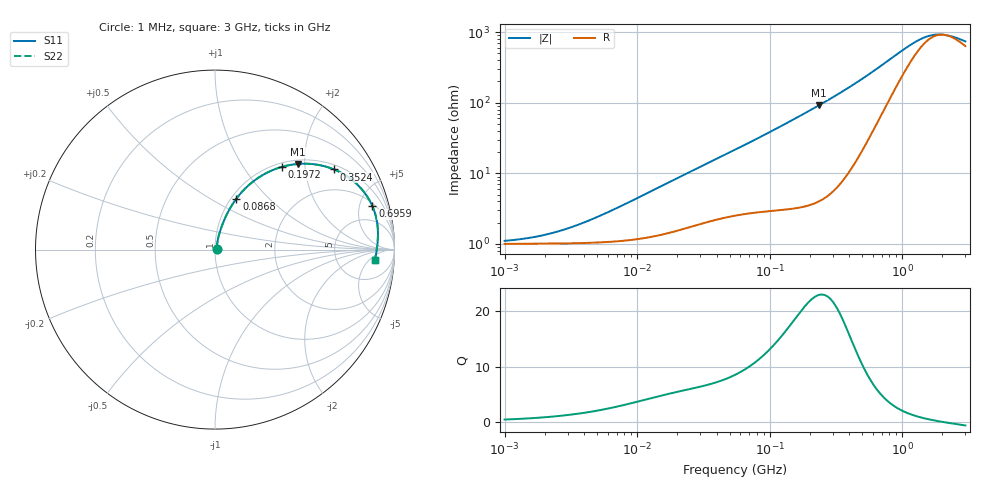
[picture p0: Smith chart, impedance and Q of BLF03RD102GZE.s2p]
! BLF03RD102GZE
# Hz S RI R 50
!Freq.(Hz) S11(Real) S11(Imag) S21(Real) S21(Imag) S12(Real) S12(Imag) S22(Real) S22(Imag)
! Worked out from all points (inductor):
!   401 points, 1 MHz to 3 GHz, reference 50 ohm
!   read as one part in series: L = 68.3 nH near 7.703 MHz
!   highest Q = 22.9 at 236.1 MHz (marker M1), where L = 61.9 nH
!   self-resonance near 2.068 GHz
!   S11 on the Smith chart (normalised r, x): 1 MHz: 1.02, +0.01; 86.8 MHz: 1.06, +0.66; 197.2 MHz: 1.07, +1.52; 352.4 MHz: 1.15, +2.86; 695.9 MHz: 2.33, +6.56; 3 GHz: 14, -8
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1000000  0.00993 0.0046  0.9901 -0.0046  0.9901 -0.0046  0.00993 0.0046
2014875  0.0101 0.00873  0.9899 -0.00873  0.9899 -0.00873  0.0101 0.00873
3823119  0.0105 0.0163  0.9895 -0.0163  0.9895 -0.0163  0.0105 0.0163
6433254  0.0114 0.0272  0.9886 -0.0272  0.9886 -0.0272  0.0114 0.0272
1.461624e7  0.0168 0.0602  0.9832 -0.0602  0.9832 -0.0602  0.0168 0.0602
3.00453e7  0.0327 0.1161  0.9673 -0.1161  0.9673 -0.1161  0.0327 0.1161
5.477226e7  0.0652 0.195  0.9348 -0.195  0.9348 -0.195  0.0652 0.195
8.679508e7  0.1195 0.2845  0.8805 -0.2845  0.8805 -0.2845  0.1195 0.2845
1.321429e8  0.2168 0.3828  0.7832 -0.3828  0.7832 -0.3828  0.2168 0.3828
1.971969e8  0.3719 0.4607  0.6281 -0.4607  0.6281 -0.4607  0.3719 0.4607
2.094008e8  0.4003 0.468  0.5997 -0.468  0.5997 -0.468  0.4003 0.468
2.361213e8  0.4599 0.477  0.5401 -0.477  0.5401 -0.477  0.4599 0.477
2.884452e8  0.5636 0.4739  0.4364 -0.4739  0.4364 -0.4739  0.5636 0.4739
3.523638e8  0.6641 0.4463  0.3359 -0.4463  0.3359 -0.4463  0.6641 0.4463
4.951867e8  0.8007 0.3548  0.1993 -0.3548  0.1993 -0.3548  0.8007 0.3548
6.958997e8  0.8769 0.2422  0.1231 -0.2422  0.1231 -0.2422  0.8769 0.2422
8.005644e8  0.8927 0.1987  0.1073 -0.1987  0.1073 -0.1987  0.8927 0.1987
1.243477e9  0.9081 0.0883  0.0919 -0.0883  0.0919 -0.0883  0.9081 0.0883
1.645649e9  0.9055 0.0363  0.0945 -0.0363  0.0945 -0.0363  0.9055 0.0363
1.855641e9  0.9035 0.0168  0.0965 -0.0168  0.0965 -0.0168  0.9035 0.0168
2.134733e9  0.9007 -0.00484  0.0993 0.00484  0.0993 0.00484  0.9007 -0.00484
3e9  0.892 -0.0555  0.108 0.0555  0.108 0.0555  0.892 -0.0555
